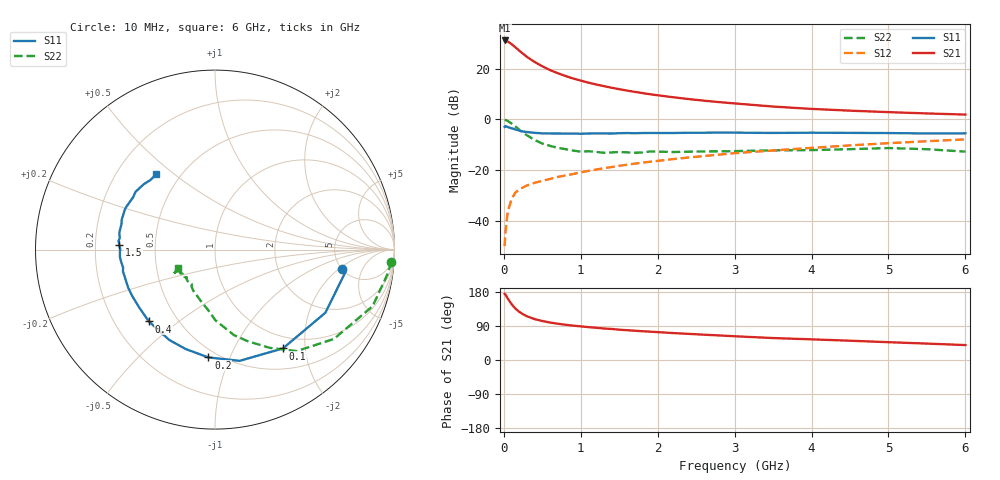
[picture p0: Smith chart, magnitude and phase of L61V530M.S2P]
!  INFINEON TECHNOLOGIES Small Signal Semiconductors
! BFR380L3 , Si-NPN RF-Transistor in TSLP-3-1
!  Vce=1.5 V,  Ic=30 mA
! Common Emitter S-Parameters:  07. March 2005
#  GHz  S  MA  R  50
! f  S11  S21  S12  S22
! GHz  Mag  Ang  Mag  Ang  Mag  Ang  Mag  Ang
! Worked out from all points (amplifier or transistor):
!   36 points, 10 MHz to 6 GHz, reference 50 ohm
!   highest |S21| = 31.1 dB at 10 MHz (marker M1)
!   |S21| within 3 dB of that: start of sweep to 161.9 MHz
!   unconditionally stable (mu >= 1): 1.816 GHz to 4.932 GHz
!   at 250 MHz: K = 0.40, MSG = 26.3 dB, |S12| = -26.7 dB
!   at 1.4 GHz: K = 0.97, MSG = 15.6 dB, |S12| = -18.8 dB
!   at 6 GHz: K = 0.98, MSG = 4.9 dB, |S12| = -7.9 dB
!   S11 on the Smith chart (normalised r, x): 10 MHz: 5.02, -2.16; 100 MHz: 0.80, -1.60; 200 MHz: 0.44, -0.84; 400 MHz: 0.35, -0.39; 1.5 GHz: 0.30, +0.02; 6 GHz: 0.37, +0.43
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0.01  0.7137 -8.5  35.77 174.6  0.0032 74.1  0.9851 -3.9
0.02  0.7384 -9.5  35.52 173.0  0.0059 81.5  0.9704 -8.2
0.05  0.7084 -29.8  34.17 162.4  0.015 76.9  0.9334 -19.7
0.1  0.668 -55.5  30.37 147.5  0.0271 66.9  0.829 -36.9
0.15  0.6348 -77.5  26.27 135.7  0.0362 59.1  0.7256 -51.2
0.2  0.6019 -93.5  22.52 127.1  0.0418 55.4  0.6273 -60.8
0.25  0.5775 -106.5  19.53 120.6  0.046 51.5  0.5424 -70.3
0.3  0.5642 -116.9  17.01 115.4  0.0502 51.3  0.4879 -77.5
0.4  0.544 -132.6  13.5 107.9  0.0565 50.4  0.3936 -89.7
0.5  0.5314 -142.8  11.11 102.9  0.0617 51.4  0.3353 -97.1
0.6  0.5288 -150.9  9.351 98.8  0.0674 52.7  0.3016 -104.4
0.7  0.5283 -156.3  8.124 95.8  0.0737 54.3  0.2758 -111.3
0.9  0.527 -166.6  6.386 90.7  0.0841 56.6  0.2432 -122.5
1.1  0.5273 -172.6  5.289 86.7  0.0969 59.0  0.2363 -128.3
1.5  0.5347 177.1  3.931 80.0  0.122 61.2  0.2282 -138.2
1.8  0.5393 171.1  3.299 75.9  0.1409 62.0  0.2232 -143.4
2.2  0.5399 164.9  2.73 71.1  0.1655 62.6  0.2281 -146.0
2.8  0.5496 156.1  2.188 64.8  0.2026 63.0  0.2348 -151.6
3.5  0.5416 147.5  1.789 57.9  0.2444 61.2  0.2458 -150.6
4.5  0.543 141.2  1.486 50.9  0.3081 59.7  0.2597 -149.9
5.5  0.529 133.0  1.31 43.3  0.3718 55.9  0.259 -150.2
6  0.5318 128.0  1.244 39.4  0.4047 53.7  0.232 -153.6
